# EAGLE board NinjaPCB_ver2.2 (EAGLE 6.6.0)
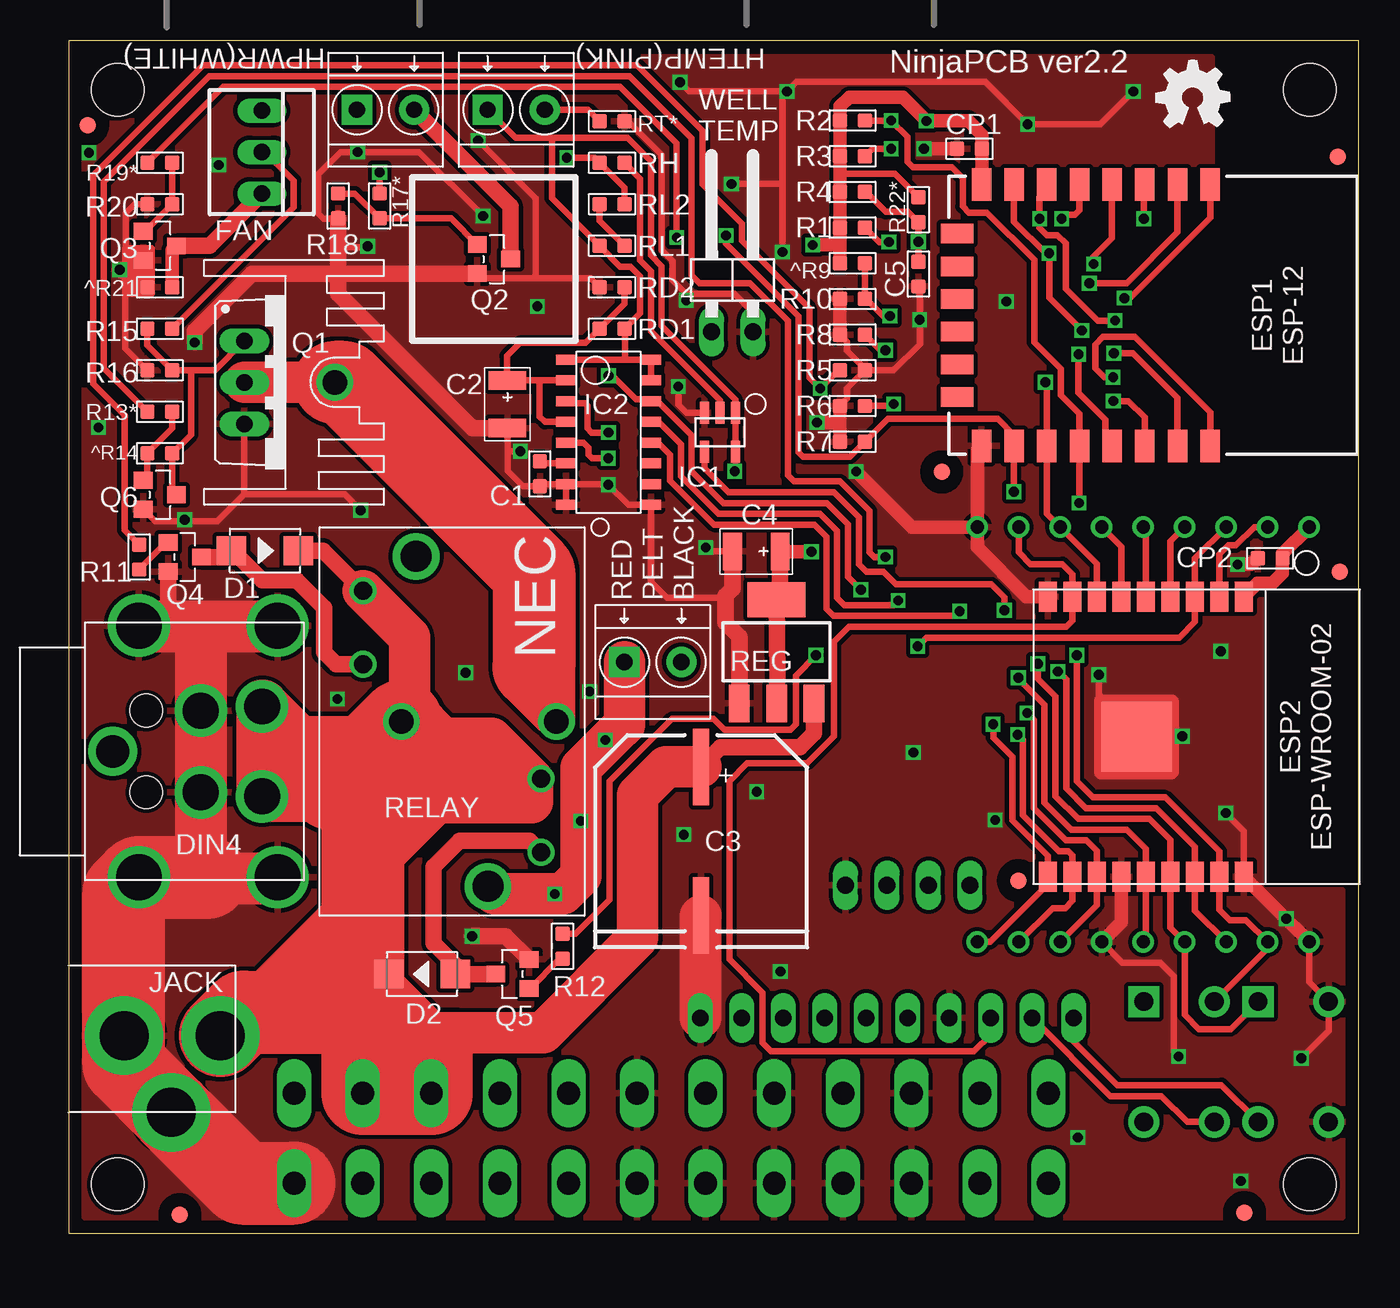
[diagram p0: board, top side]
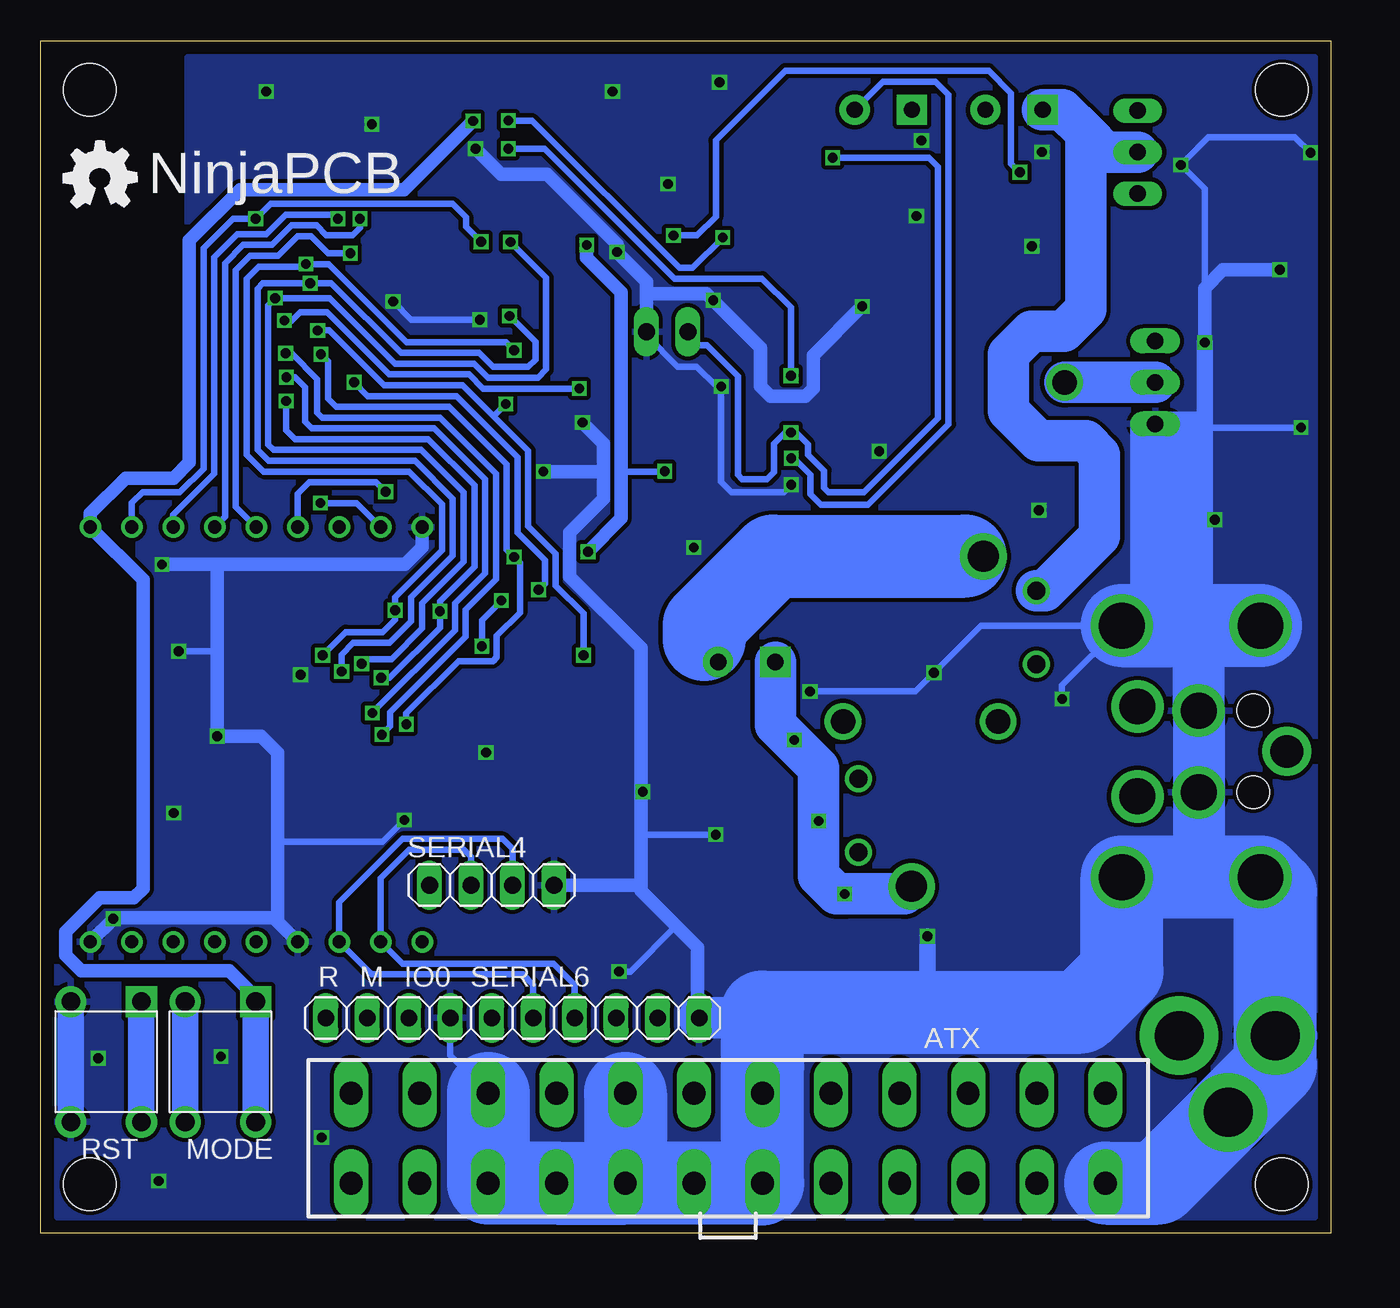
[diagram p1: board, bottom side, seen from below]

Size 79 x 73 mm. Coordinates in mm from the lower left corner, seen from the top.
Outline: 0,0 79,0 79,73 0,73 0,0
Copper layers (1*16): Top 0.035mm / dielectric 1.5mm / Bottom 0.035mm
Design rules "SeeedStudio_2oz": minimum track width 6mil, minimum drill 12mil, track to track 10mil, track to pad 10mil, pad to pad 10mil, via to via 10mil, smd to smd 0mil, copper to edge 10mil, drill to drill 10mil, minimum pad ring 10mil, minimum via ring 6mil, stop-mask expansion 2mil, vias tented up to drill 100mil, thermal gap 10mil
Net classes: 1 2A: width 0.406 mm; 2 8A: width 2.54 mm
Holes 3.2 mm at 3,3 3,70 76,70 76,3
tKeepout: area 1.4,1.4 to 4.6,4.6; area 74.4,1.4 to 77.6,4.6; area 74.4,68.4 to 77.6,71.6; area 1.4,68.4 to 4.6,71.6

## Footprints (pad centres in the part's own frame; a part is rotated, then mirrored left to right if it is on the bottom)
ATX24 = drill 1.4 long: 1 23.1,-2.75; 2 18.9,-2.75; 3 14.7,-2.75; 4 10.5,-2.75; 5 6.3,-2.75; 6 2.1,-2.75; 7 -2.1,-2.75; 8 -6.3,-2.75; 9 -10.5,-2.75; 10 -14.7,-2.75; 11 -18.9,-2.75; 12 -23.1,-2.75; 13 23.1,2.75; 14 18.9,2.75; 15 14.7,2.75; 16 10.5,2.75; 17 6.3,2.75; 18 2.1,2.75; 19 -2.1,2.75; 20 -6.3,2.75; 21 -10.5,2.75; 22 -14.7,2.75; 23 -18.9,2.75; 24 -23.1,2.75
C0603 = smd 0.889 x 0.889: 1 0,0.762; 2 0,-0.762
AVX-B = smd 1.143 x 2.286: + -1.46,0; - 1.46,0
CAP_SMD_AL_D125 = smd 1 x 4.7: P$M 0,-4.55; P$P 0,4.55
DO-214AC = smd 1.8 x 1.77: 1 -2.042,0; 2 2.042,0
DIN4 = drill 2.2: P$1 -2.75,10.85; P$2 2.75,10.85; P$3 -2.5,7.1; P$4 2.5,7.1 | drill 2: P$5 0,1.7 | drill 2.8: P$6 -7.7,11.8; P$7 -7.7,3.3; P$8 7.7,3.3; P$9 7.7,11.8 | hole 2: -2.5,3.75; 2.5,3.75
ESP-12F = smd 2 x 1.2: 1 -8,3.48; 2 -8,1.48; 3 -8,-0.52; 4 -8,-2.52; 5 -8,-4.52; 6 -8,-6.52; 7 -8,-8.52; 8 -8,-10.52; 15 8,-10.52; 16 8,-8.52; 17 8,-6.52; 18 8,-4.52; 19 8,-2.52; 20 8,-0.52; 21 8,1.48; 22 8,3.48 | smd 1.2 x 2: 9 -5,-12; 10 -3,-12; 11 -1,-12; 12 1,-12; 13 3,-12; 14 5,-12
ESP-WROOM-02 = smd 1.85 x 1.1: P$1 -8.575,12.9; P$2 -8.575,11.4; P$3 -8.575,9.9; P$4 -8.575,8.4; P$5 -8.575,6.9; P$6 -8.575,5.4; P$7 -8.575,3.9; P$8 -8.575,2.4; P$9 -8.575,0.9; P$10 8.575,0.9; P$11 8.575,2.4; P$12 8.575,3.9; P$13 8.575,5.4; P$14 8.575,6.9; P$15 8.575,8.4; P$16 8.575,9.9; P$17 8.575,11.4; P$18 8.575,12.9 | smd 4.3 x 4.3: P$19 0,6.33
ESP-WROOM-02-BREAK-NODETAIL = drill 0.8: P$1 -12.7,10.16; P$2 -12.7,7.62; P$3 -12.7,5.08; P$4 -12.7,2.54; P$5 -12.7,0; P$6 -12.7,-2.54; P$7 -12.7,-5.08; P$8 -12.7,-7.62; P$9 -12.7,-10.16; P$10 12.7,-10.16; P$11 12.7,-7.62; P$12 12.7,-5.08; P$13 12.7,-2.54; P$14 12.7,0; P$15 12.7,2.54; P$16 12.7,5.08; P$17 12.7,7.62; P$18 12.7,10.16
22-23-2031 = drill 1 long: 1 -2.54,0; 2 0,0; 3 2.54,0
H2-3.5-7.0X7.0MM = drill 1 pad 1.85 square: 1 -1.75,0 | drill 1 pad 1.85: 2 1.75,0
HEAT11PB015 = drill 1.5: P$1 0,3
SOT23-5 = smd 1.321 x 0.559: 1 -1.194,0.95; 2 -1.194,0; 3 -1.194,-0.95; 4 1.194,-0.95; 6 1.194,0.95
SOP-16 = smd 0.6 x 1.2: P$1 -4.445,-2.6; P$2 -3.175,-2.6; P$3 -1.905,-2.6; P$4 -0.635,-2.6; P$5 0.635,-2.6; P$6 1.905,-2.6; P$7 3.175,-2.6; P$8 4.445,-2.6; P$9 4.445,2.6; P$10 3.175,2.6; P$11 1.905,2.6; P$12 0.635,2.6; P$13 -0.635,2.6; P$14 -1.905,2.6; P$15 -3.175,2.6; P$16 -4.445,2.6
1X02 = drill 1.016 long: 1 -1.27,0; 2 1.27,0
PJ-102A-NOOUT = drill 3 pad 4.8: RING 0.1,-3.39; RING_SW -4.6,-6.29; TIP 0.1,-9.29
SW4-6.0X6.0X5.0MM = drill 1.143 pad 1.905 square: 1 -3.683,2.159 | drill 1.143 pad 1.905: 2 -3.683,-2.159; 3 3.683,-2.159; 4 3.683,2.159
TO220BV = drill 1.016 long: D 0,-2.54; G -2.54,-2.54; S 2.54,-2.54
SOT-23 = smd 1.016 x 1.143: 1 -0.889,-1.016; 2 0.889,-1.016; 3 0,1.016
R0603 = smd 0.889 x 0.889: 1 0,0.762; 2 0,-0.762
SOT-223 = smd 1.27 x 2.286: 1 -2.286,-3.175; 2 0,-3.175; 3 2.286,-3.175 | smd 3.556 x 2.159: TER 0,3.175
NEC-EP2 = drill 1.9: P$1 -10.1,-2.2; P$8 10.1,2.2 | drill 1.1: P$2 -8,-5.45; P$3 -3.5,-5.45; P$6 3.5,5.45; P$7 8,5.45 | drill 1.5: P$4 0,-3.1; P$5 0,6.4
1X04 = drill 1.016 long: 1 -3.81,0; 2 -1.27,0; 3 1.27,0; 4 3.81,0
1X06 = drill 1.016 long: 1 -6.35,0; 2 -3.81,0; 3 -1.27,0; 4 1.27,0; 5 3.81,0; 6 6.35,0
FIDUCIAL_1MM = smd 1 x 1: 1 0,0
1X02/90 = drill 1.016 long: 1 -1.27,-3.81; 2 1.27,-3.81

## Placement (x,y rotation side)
ATX  ATX24NH  [ATX24]  36.91,5.82 180 bottom
C1  100nf  [C0603]  28.86,46.49 180 top
C2  22uf  [AVX-B]  26.87,50.75 270 top
C3  CAP_SMDAL_1000UF_25V  [CAP_SMD_AL_D125]  38.73,24 0 top
C4  22uf  [AVX-B]  42.11,41.74 180 top
C5  100nf  [C0603]  52.04,58.72 180 top
CP1  100nf  [C0603]  55.16,66.4 270 top
CP2  100nf  [C0603]  73.57,41.32 90 top
D1  1N4007  [DO-214AC]  12.02,41.79 0 top
D2  1N4007  [DO-214AC]  21.64,15.88 180 top
DIN4  [DIN4]  1,29.5 270 top
ESP1  ESP-12F  [ESP-12F]  66.42,56.2 270 top
ESP2  ESP-WROOM-02  [ESP-WROOM-02]  59.08,30.4 270 top
ESP3  ESP-WROOM-02-BREAKND  [ESP-WROOM-02-BREAK-NODETAIL]  65.8,30.54 270 top
FAN  22-23-2031  [22-23-2031]  11.83,66.19 270 top
HEATER_POWER  [H2-3.5-7.0X7.0MM]  19.41,68.78 0 top
HEATER_TEMP  [H2-3.5-7.0X7.0MM]  27.41,68.78 0 top
HEATSINK  HEAT111PB015  [HEAT11PB015]  13.3,52.09 270 top
IC1  ANALOGSW_AD_SOT23-5  [SOT23-5]  39.88,49.04 270 top
IC2  NAU7802  [SOP-16]  33.06,49.04 270 top
IO0  [1X02]  55.19,13.18 0 bottom
JACK  2.1MMJACKTHM-NOOUT  [PJ-102A-NOOUT]  0,12 90 top
MODE  [SW4-6.0X6.0X5.0MM]  68,10.5 270 bottom
PELTIER  [H2-3.5-7.0X7.0MM]  35.77,34.97 0 top
Q1  IRLB3813PBF  [TO220BV]  13.3,52.09 270 top
Q2  CJ2302  [SOT-23]  26.04,59.63 270 top
Q3  CJ2302  [SOT-23]  5.59,60.45 270 top
Q4  S9013  [SOT-23]  7.11,41.4 270 top
Q5  S9013  [SOT-23]  27.18,15.88 90 top
Q6  S9013  [SOT-23]  5.59,45.21 270 top
R1  10K 1/10W  [R0603]  48.01,61.57 90 top
R2  10K 1/10W  [R0603]  48.01,68.12 90 top
R3  10K 1/10W  [R0603]  48.01,65.94 90 top
R4  10K 1/10W  [R0603]  48.01,63.75 90 top
R5  10K 1/10W  [R0603]  48.01,52.83 270 top
R6  10K 1/10W  [R0603]  48.01,50.65 90 top
R7  10K 1/10W  [R0603]  48.01,48.46 90 top
R8  10K 1/10W  [R0603]  48.01,55.02 90 top
R9  100K 1/10W  [R0603]  48.01,59.39 270 top
R10  10K 1/10W  [R0603]  48.01,57.2 270 top
R11  10K 1/10W  [R0603]  4.32,41.4 0 top
R12  10K 1/10W  [R0603]  30.25,17.58 180 top
R13  1K 1/10W  [R0603]  5.59,50.29 90 top
R14  0R  [R0603]  5.59,47.75 90 top
R15  10K 1/10W  [R0603]  5.59,55.37 90 top
R16  10K 1/10W  [R0603]  5.59,52.83 90 top
R17  1K 1/10W  [R0603]  19.05,62.89 0 top
R18  10K 1/10W  [R0603]  16.51,62.89 180 top
R19  1K 1/10W  [R0603]  5.59,65.53 90 top
R20  10K 1/10W  [R0603]  5.59,62.99 90 top
R21  0R  [R0603]  5.59,57.91 90 top
R22  1K 1/10W  [R0603]  52.04,62.66 180 top
RD1  15K HP  [R0603]  33.27,55.37 90 top
RD2  15K HP  [R0603]  33.27,57.91 270 top
REG  CJT1117-3.3-SOT223  [SOT-223]  43.36,35.61 0 top
RELAY  NEC-RELAY2EP2  [NEC-EP2]  23.48,31.34 270 top
RESET  [1X02]  60.27,13.18 0 bottom
RH  15K HP  [R0603]  33.27,65.53 270 top
RL1  15K HP  [R0603]  33.27,60.45 90 top
RL2  15K HP  [R0603]  33.27,62.99 90 top
RST  [SW4-6.0X6.0X5.0MM]  75,10.5 270 bottom
RT  4.99K HP  [R0603]  33.27,68.07 90 top
SERIAL4  [1X04]  51.38,21.31 0 bottom
SERIAL6  [1X06]  45.03,13.18 0 bottom
U$1  [OSHW_5MM]  68.83,69.52 0 top
U$2  [OSHW_5MM]  75.39,64.59 0 bottom
U$3  FIDUCIAL  [FIDUCIAL_1MM]  77.72,65.91 270 top
U$4  FIDUCIAL  [FIDUCIAL_1MM]  6.81,1.14 0 top
U$5  FIDUCIAL  [FIDUCIAL_1MM]  72.01,1.27 0 top
U$7  FIDUCIAL  [FIDUCIAL_1MM]  1.17,67.84 0 top
U$8  FIDUCIAL  [FIDUCIAL_1MM]  58.17,21.59 270 top
U$9  FIDUCIAL  [FIDUCIAL_1MM]  53.47,46.61 270 top
U$10  FIDUCIAL  [FIDUCIAL_1MM]  77.85,40.51 270 top
WELL_TEMP  [1X02/90]  40.64,59 0 top

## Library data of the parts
ATX DIN4 HEATSINK = PCR-Connector
C1 C5 CP1 CP2 = Seeed-Capacitor; MPN: CC0603KRX7R9BB104
C2 C4 = Seeed-Capacitor; MPN: TAJB226*016#NJ
C3 = Seeed-OPL-2017-01-Capacitor-akita
D1 D2 = Seeed-Diode; MPN: 1N4007
ESP1 = Seeed-OPL-2017-01-Sensor-camilo
ESP2 ESP3 = PCR-Module
FAN = con-molex; MF: MOLEX; MPN: 22-23-2031; OC_FARNELL: 1462950; OC_NEWARK: 30C0862
HEATER_POWER HEATER_TEMP PELTIER = Seeed-Connector
IC1 IC2 = PCR-IC
IO0 RESET SERIAL4 SERIAL6 WELL_TEMP = pinhead
JACK U$3-U$5 U$7-U$10 = adafruit
MODE RST = Seeed-Switch
Q1 = transistor-power
Q2 Q3 = Seeed-Transistor; MPN: CJ2302
Q4-Q6 = Seeed-Transistor; MPN: S9013
R1-R8 R10-R12 R15 R16 R18 R20 = Seeed-Resistor; MPN: RC0603JR-0710KL
R9 = Seeed-Resistor; MPN: RC0603JR-07100KL
R13 R17 R19 R22 = Seeed-Resistor; MPN: RC0603JR-071KL
R14 R21 = Seeed-Resistor; MPN: RC0603JR-070RL
RD1 RD2 RH RL1 RL2 = PCR-RCL
REG = Seeed-IC; MPN: CJT1117-3.3
RELAY = PCR-Switch
RT = Seeed-Resistor; MPN: RC0603FR-072KL
U$1 U$2 = oshw

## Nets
3V3: C4.+ CP1.1 CP2.2 ESP1.8 ESP2.P$1 ESP3.P$1 HEATER_TEMP.1 IC1.1 IC1.6 IC2.P$1 IC2.P$15 IC2.P$16 MODE.1 MODE.4 R1.1 R2.1 R3.1 R4.1 R9.2 R22.2 RD1.2 REG.2 REG.TER RL1.1
12V: ATX.10 ATX.11 C3.P$P D1.2 D2.2 DIN4.P$1 DIN4.P$2 FAN.2 HEATER_POWER.1 JACK.TIP R15.2 REG.3 RELAY.P$2 RELAY.P$4 RELAY.P$6
BLK: PELTIER.2 RELAY.P$1
DIVIDED: C2.+ IC2.P$2 IC2.P$4 RD1.1 RD2.1
DRDY: ESP1.20 ESP2.P$14 ESP3.P$14 IC2.P$12
EN: C5.2 ESP1.3 ESP2.P$2 ESP3.P$2 R4.2 R22.1
FAN: ESP1.18 ESP2.P$8 ESP3.P$8 IO0.1 R2.2 R19.1
GND: ATX.3 ATX.5 ATX.7 ATX.15 ATX.16 ATX.17 ATX.18 ATX.19 ATX.24 C1.1 C2.- C3.P$M C4.- C5.1 CP1.2 CP2.1 DIN4.P$3 DIN4.P$4 DIN4.P$6 DIN4.P$7 DIN4.P$8 DIN4.P$9 ESP1.15 ESP2.P$9 ESP2.P$13 ESP2.P$18 ESP2.P$19 ESP3.P$9 ESP3.P$13 ESP3.P$18 IC1.3 IC2.P$7 IC2.P$8 IC2.P$9 IO0.2 JACK.RING JACK.RING_SW Q1.S Q2.2 Q3.2 Q4.2 Q5.2 Q6.2 R5.1 R6.1 R7.1 R8.1 R10.2 R16.1 R18.1 R20.1 R21.1 RD2.2 REG.1 RST.2 RST.3 RT.2 SERIAL4.4 SERIAL6.6 WELL_TEMP.2
HEATER: ESP1.16 ESP2.P$6 ESP3.P$6 R7.2 R17.1
HEATER_TEMP: HEATER_TEMP.2 IC2.P$5 RT.1
HIGH_TEMP: ESP1.4 ESP2.P$17 ESP3.P$17 IC1.4 MODE.2 MODE.3 R8.2 RESET.2
N$1: RL1.2 RL2.1
N$2: HEATER_POWER.2 Q2.3
N$3: HEATSINK.P$1 Q1.D RELAY.P$5
N$4: FAN.3 Q3.3 R21.2
N$5: Q1.G Q6.3 R14.2 R15.1 R16.2
N$8: Q3.1 R19.2 R20.2
N$27: IC1.2 RH.1
N$30: Q6.1 R13.2 R14.1
N$32: Q2.1 R17.2 R18.2
N$33: D1.1 Q4.3 RELAY.P$3
N$34: Q4.1 R11.2
N$35: Q5.1 R12.1
N$36: D2.1 Q5.3 RELAY.P$7
N$92: C1.2 IC2.P$6
PEL_PWM: ESP1.19 ESP2.P$10 ESP3.P$10 R13.1
PEL_SWA: ESP1.6 ESP2.P$4 ESP3.P$4 R5.2 R11.1
PEL_SWB: ESP1.7 ESP2.P$5 ESP3.P$5 R6.2 R12.2
RED: PELTIER.1 RELAY.P$8
RESET: ESP1.1 ESP2.P$15 ESP3.P$15 R1.2 RESET.1 RST.1 RST.4
RXD: ESP1.21 ESP2.P$11 ESP3.P$11 SERIAL4.2 SERIAL6.3
SCLK: ESP1.5 ESP2.P$3 ESP3.P$3 IC2.P$13
SDIO: ESP1.17 ESP2.P$7 ESP3.P$7 IC2.P$14 R3.2
TOUT: ESP1.2 ESP2.P$16 ESP3.P$16 R9.1 R10.1
TXD: ESP1.22 ESP2.P$12 ESP3.P$12 SERIAL4.3 SERIAL6.2
WELL_TEMP: IC2.P$3 RH.2 RL2.2 WELL_TEMP.1

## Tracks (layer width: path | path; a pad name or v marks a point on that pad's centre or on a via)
3V3  (via drill 0.6)
  Top 0.406: IC2.P$1 34.09,53.48 | 34.09,53.48 IC2.P$16 IC2.P$15 | 34.09,53.48 34.09,55.32 RD1.2 35,56.34 35,58.6 34.42,59.18 33.78,59.18 RL1.1 29.59,63.37 29.59,67.08 | HEATER_TEMP.1 27.36,67.08 29.59,67.08 | 29.59,67.08 34.21,67.08 35.66,65.63 35.66,59.87 36.32,59.21 36.32,55.55 40.83,51.04 IC1.1 IC1.6 40.83,46.66 v40.79,46.66 | R22.2 50.6,64.87 47.24,64.87
  Top 0.813: 43.35,34.1 43.41,34.16 | C4.+ 43.66,41.73 v45.49,41.73 | ESP1.8 55.93,64.2 CP1.1 55.93,67.26 55.09,68.1 v52.53,68.1 51.08,69.55 47.8,69.55 47.24,68.99 R2.1 R3.1 47.24,64.87 R4.1 R1.1 47.24,60.5 | ESP2.P$1 72.8,39.8 73.71,39.8 74.31,40.4 CP2.2 74.34,41.61 ESP3.P$1 | v45.57,60.5 47.24,60.5 | R9.2 47.24,60.5
  Top 1.016: REG.2 43.41,34.16 REG.TER 43.58,39.01 C4.+
  Bottom 0.406: 45.49,41.83 v45.49,41.73 | v40.79,46.66 40.82,46.63 43.46,46.63
  Bottom 0.813: v45.49,41.73 43.46,43.76 43.46,46.63 43.46,57.61 45.57,59.72 v45.57,60.5 | MODE.1 65.84,14.46 67.46,16.08 76.53,16.08 77.47,17.02 77.47,18.47 75.39,20.55 73.3,20.55 72.75,21.11 72.75,40.02 ESP3.P$1 75.96,44.08 73.81,46.23 70.87,46.23 69.9,47.19 69.9,60.78 66.8,63.88 56.74,63.88 v52.53,68.1
  Bottom 1.626: MODE.4 MODE.1
12V
  Top 0.254: 28.37,27.84 28.36,27.84 28.36,27.85 | 19.25,15.21 20.4,15.21 20.4,12.29 | 17.2,20.02 18.01,20.02 18.01,20.24
  Top 0.406: FAN.2 12.05,66.19 13.79,64.44 13.79,62.81 R15.2 | DIN4.P$1 11.86,32.26 | 23.5,8.56 22.22,8.56 ATX.10
  Top 0.508: 16.05,27.23 16.48,27.23 16.71,27.46
  Top 1.016: RELAY.P$2 15.58,41.79 D1.2 | D2.2 19.53,15.74 17.32,13.54 17.5,13.36 17.5,12.9 18.01,12.39 ATX.11 | REG.3 45.65,30.61 44.78,29.74 39.91,29.74 C3.P$P
  Top 1.27: 28.37,27.84 RELAY.P$6
  Top 2.54: RELAY.P$2 20.88,36.49 20.88,32.21 20.38,31.71 RELAY.P$4 23.88,27.84 28.37,27.84 | 23.72,12.29 23.5,12.06 23.5,8.56 | 23.72,12.29 20.4,12.29 | 23.72,12.29 29.06,12.29 34.85,18.09 34.85,26.82 36.58,28.55 C3.P$P | 18.62,20.75 18.62,22.45 23.39,27.23 21.06,27.23 20.75,26.92 20.75,27.64 21.34,28.22 23.19,26.36 28.35,26.36 28.4,26.42 28.4,27.81 28.36,27.85 25.91,30.3 22.91,30.3 21.08,32.13 20.73,32.13 19,30.4 14.02,30.4 | 19.25,21.39 19.25,15.21 21.89,12.57 | 17.2,23.27 17.2,20.02 12.06,14.88 14.55,14.88 15.6,15.93
  Top 3.175: 15.36,26.75 DIN4.P$2 DIN4.P$1 | 11.89,32.23 11.86,32.26 11.86,32.31 16.71,27.46 | 13.01,28.73 13.56,28.17 14.15,28.17
  Top 5.08: ATX.10 ATX.11 18.01,20.24 18.01,26.16 16.71,27.46 | RELAY.P$4 16.27,27.23 16.05,27.23 15.11,28.17 14.15,28.17 | JACK.TIP 10.73,13.54 17.32,13.54 17.45,13.54
  Bottom 2.54: 15.01,67.36 15.01,56.57 16.36,55.22 18.34,55.22 19.74,53.82 19.74,50.34 17.91,48.51 15.01,48.51 14.17,47.68 14.17,42.67 17.51,39.34 RELAY.P$2 | 15.01,67.36 16.43,68.78 HEATER_POWER.1 | 15.01,67.36 13.84,66.19 FAN.2
BLK
  Bottom 0.508: 38.38,36.35 37.52,35.49 PELTIER.2 | 22.4,41.45 22.39,41.44 RELAY.P$1
  Bottom 5.08: 38.38,36.35 38.38,37.24 34.16,41.45 22.4,41.45
DIVIDED
  Top 0.406: IC2.P$2 28.8,52.21 | 28.8,52.21 C2.+ 26.85,52.24 26.85,53.72 27.64,54.51 31.65,54.51 RD1.1 34.04,56.9 RD2.1 | IC2.P$4 29.17,49.67 28.85,49.99 28.85,52.16 28.8,52.21
DRDY  (via drill 0.6)
  Top 0.406: IC2.P$12 36.1,48.4 36.83,47.68 36.83,46.08 39.52,43.38 45.67,43.38 46.41,42.65 46.41,38.23 46.84,37.8 54.28,37.8 v54.56,38.08 | ESP3.P$14 65.98,18.01 ESP2.P$14 65.98,23.53 64.8,24.71 61.42,24.71 59.77,26.36 59.77,32.36 58.17,33.96 v58.17,34.01 | ESP1.20 65.9,49.95 64.9,50.95 v63.98,50.95
  Bottom 0.406: v63.98,50.95 63.98,49.17 63.42,48.62 55.27,48.62 52.45,45.8 52.45,40.79 54.56,38.68 v54.56,38.08 54.56,37.08 57.63,34.01 v58.17,34.01
EN  (via drill 0.6)
  Top 0.406: ESP2.P$2 70.48,41.57 71.02,42.11 71.48,42.11 72.6,43.24 ESP3.P$2 | ESP1.3 65.84,64.14 v65.84,62.1 | R4.2 48.82,63.75 50.04,62.53 51.41,62.53 R22.1 v52.05,60.69 C5.2
  Bottom 0.406: ESP3.P$2 73.42,44.71 72.77,45.36 70.48,45.36 69.04,46.81 69.04,60.3 67.23,62.1 v65.84,62.1 64.92,63.02 53.77,63.02 52.96,62.2 52.96,61.61 v52.05,60.69
FAN  (via drill 0.6)
  Top 0.406: R19.1 9.47,70.18 33.78,70.18 37.24,66.73 v37.24,60.96 | ESP3.P$8 58.18,41.69 58.9,40.97 60.86,40.97 61.48,40.35 ESP2.P$8 61.48,37.5 61.11,37.13 47.78,37.13 46.86,36.22 46.86,30.43 45.21,28.78 41.55,28.78 40.46,27.69 40.46,16.76 42.49,14.73 42.49,11.66 43,11.15 55.45,11.15 56.46,12.17 IO0.1 | v61.87,44.7 61.9,44.73 ESP1.18 61.9,50.16 60.76,51.31 60.76,52.93 59.13,54.56 59.13,59.59 56.24,62.48 55.14,62.48 54.76,62.87 54.76,64.59 54.1,65.25 51.71,65.25 51.36,65.61 51.36,67.13 v50.37,68.12 R2.2
  Bottom 0.406: ESP3.P$8 59.65,44.7 v61.87,44.7 | v37.24,60.96 39.09,59.11 39.9,59.11 48.92,68.12 v50.37,68.12
GND  (via drill 0.6)
  Top 0.406: Q6.2 5.31,43.59 7.01,43.59 | 7.01,43.59 9.09,43.59 10.76,45.26 | 10.76,45.26 Q1.S | 4.83,59.31 Q3.2 | R20.1 4.04,62.99 3.5,62.46 3.5,60.33 | 4.29,59.56 Q3.2 | 3.5,60.33 4.06,59.77 4.37,59.77 Q3.2 | R21.1 4.8,57.91 4.78,57.89 | 5.08,58.42 5.08,57.53 3.48,57.53 | 3.48,57.53 3.48,60.3 | 3.48,60.3 3.76,60.3 3.76,59.38 3.79,59.38 3.79,60.3 5.08,60.3 5.08,59.74 4.01,59.74 4.01,60.07 4.57,60.07 4.57,60.05 | IC2.P$8 IC2.P$7 | IC2.P$7 28.99,45.86 C1.1 27.83,45.73 26.87,46.69 26.87,47.88 | 26.87,47.88 C2.- | RD2.2 31.95,58.47 28.6,58.47 | 28.6,58.47 25.3,58.47 Q2.2 | IC2.P$7 33,45.86 v33.05,45.82 34.27,44.59 IC2.P$9 35.66,39.9 36.65,38.91 40.11,38.91 40.23,39.04 | v37.34,51.84 37.34,51.33 37.34,50.93 37.34,50.72 37.83,50.23 IC1.3 | RT.2 34.27,68.07 36.32,66.02 36.32,60.2 36.98,59.54 36.98,58.34 37.82,57.51 38.1,57.51 | 38.1,57.51 40.77,57.51 41.91,56.36 WELL_TEMP.2 | ESP3.P$18 75.96,15.38 RST.2 77.16,12.39 v75.49,10.72 | 4.32,21.79 5.49,21.79 5.56,21.72 | 63.25,28.19 65.96,28.19 v68.2,30.43 | 3.76,58.75 3.66,58.75 | 3.48,60.3 3.5,60.33 | 47.24,57.05 R10.2 | v18.31,60.43 18.26,60.38 16.51,60.38 | v43.99,69.9 43.71,69.62 43.71,64.24 | 43.71,64.24 v43.71,60.07 | v43.99,69.9 44.58,70.48 56.13,70.48 v58.73,67.89 63.2,67.89 v65.2,69.9 | v70.87,25.73 71.98,24.62 ESP2.P$18 | v63.09,34.19 63.09,32.31 64.19,31.22 64.59,31.22 ESP2.P$19 | v17.88,44.27 16.9,45.26 10.76,45.26 | v40.59,64.24 43.71,64.24 | v74.57,19.25 74.55,19.25 74.05,19.75 | v37.82,57.12 37.82,57.23 38.1,57.51 | R18.1 16.48,62.1 15.62,62.1 15.29,62.43 15.29,64.82 16.66,66.19 v17.7,66.19 21.46,66.19 v25.38,62.28 | v25.07,66.9 28.6,63.37 28.6,58.47
  Top 0.406: v27.66,47.88 26.87,47.88 | v39.01,41.99 39.26,41.74 C4.- | 7.01,43.59 v7.11,43.69 | v43.99,69.9 38,69.9 v37.44,70.46 | R16.1 3.48,54.18 3.48,57.53 | v67.97,10.82 67.67,11.12 67.67,15.75 66.85,16.56 64.54,16.56 ESP3.P$13 | R5.1 48.77,52.93 47.68,54.03 47.68,54.59 R8.1 | R6.1 47.68,51.08 47.68,51.74 R5.1 | R5.1 50.52,52.83 52.12,54.43 v52.12,55.93 52.12,57.89 C5.1
  Top 0.813: 4.78,57.89 3.96,57.89 3.66,58.19 3.66,58.75 4.19,58.22 4.88,58.22 4.67,58.42 4.67,59.08 4.88,58.88 | 4.88,58.88 4.88,58.29 | 4.88,58.88 4.88,59.82 | ESP2.P$9 58.66,38.98 55.64,41.99 ESP3.P$9 | CP2.1 72.43,40.95 v71.58,40.95 | ESP2.P$19 68.17,30.4 v68.2,30.43 | ESP2.P$13 64.48,19.05 ESP3.P$13 | ESP2.P$18 74.05,19.75 ESP3.P$18 | 63.25,32.59 63.27,32.56 67.56,32.56 67.59,32.54 67.59,28.25 67.54,28.19 63.25,28.19 63.22,28.22 63.22,32.59 | ESP3.P$9 55.64,47.94 ESP1.15 | v48.23,46.63 51.63,43.24 ESP3.P$9 | 47.14,57.2 R10.2 R8.1 | R7.1 47.24,49.84 | 47.24,49.84 R6.1 | v45.82,49.63 47.04,49.63 47.24,49.84 | CP1.2 v52.38,66.39 v52.38,66.4
  Top 1.016: 4.47,37.13 4.41,37.2 DIN4.P$7 5.51,37.2 6.1,37.78 Q4.2 | v3.12,58.98 3.76,58.75 Q3.2 | Q2.2 16.43,58.75 | 16.43,58.75 11.25,58.75 7.72,55.22 v7.72,54.53 | R18.1 16.51,60.38 16.51,58.82 | 16.51,58.82 16.43,58.75 | C2.- 24.75,49.29 16.51,57.53 16.51,58.82 | v24.71,18.19 26.77,18.19 Q5.2 | REG.1 41.07,36.52 40.23,37.36 40.23,39.04 40.65,39.46 C4.-
  Top 2.54: C3.P$M 38.68,19.41 SERIAL6.6
  Top 3.175: 4.19,21.77 4.24,21.72 5.56,21.72 8.1,21.72 | 12.72,21.72 8.1,21.72 | 8.1,21.72 8.1,37.13 4.47,37.13 4.24,37.13 4.24,37.16 12.85,37.16
  Top 5.08: 4.12,21.61 DIN4.P$8 4.32,21.79 | 4.32,21.79 8.46,21.79 | 4.32,21.79 3.38,20.85 3.38,10.34 6.29,7.43 JACK.RING_SW 10.62,3.07 ATX.24
  Bottom 0.254: 11.02,49.02 12.17,49.02 12.17,49.58 10.76,49.58 | 10.76,49.58 Q1.S | 9.63,49.58 10.76,49.58
  Bottom 0.406: WELL_TEMP.2 41.91,54.97 40.01,53.06 38.84,53.06 37.62,51.84 v37.34,51.84 37.34,46 36.7,45.36 33.5,45.36 v33.05,45.82 | IO0.2 53.92,10.89 ATX.3 | ATX.7 34.8,8.58 34.8,10.24 | 13.79,3.07 ATX.24 | v7.72,54.53 7.72,63.93 v9.2,65.41 7.49,67.11 2.21,67.11 v1.25,66.14 | v70.56,35.64 68.56,35.64 68.2,35.99 | v1.83,49.33 7.7,49.33 7.8,49.23 | v37.67,24.41 42.24,24.41 | v42.14,27.03 42.14,26.98 42.24,26.87 | v31.9,33.17 25.45,33.17 v24.31,34.31 21.42,37.2 DIN4.P$6 16.46,33.54 v16.46,32.72 | v43.59,16.03 42.9,16.03 40.09,18.83 | 64.49,23.98 58.06,23.98 v56.74,25.3 | v52.12,55.93 56.31,55.93 v57.43,57.05
  Bottom 0.813: v71.58,40.95 68.38,40.95 | 68.38,40.95 56.69,40.95 55.64,41.99 ESP3.P$9 | 68.38,40.95 68.2,40.77 68.2,35.99 v68.2,30.43 65.51,30.43 64.49,29.41 64.49,23.98 64.49,19.07 | ESP3.P$13 64.49,19.07 | 64.49,19.07 64.75,19.33 74.47,19.33 ESP3.P$18 | 44.53,46.81 44.53,44.98 46.61,42.9 46.61,40.21 42.24,35.84 42.24,26.87 42.24,24.41 42.24,21.31 | v48.23,46.63 44.65,46.63 44.53,46.81 | WELL_TEMP.2 41.91,57.68 | 41.91,57.68 41.91,58.27 v43.71,60.07 43.71,60.55 48.01,64.85 50.83,64.85 v52.38,66.4 | 34.8,3.07 ATX.19 35.2,3.47 35.2,12.9 35.46,13.16 38.71,13.16 38.79,13.23 38.79,17.53 40.09,18.83 42.24,20.98 42.24,21.31 | SERIAL4.4 42.24,21.31 | v28.7,56.74 31.7,53.75 31.7,51.74 32.18,51.26 34.31,51.26 34.92,51.87 34.92,54.2 38.23,57.51 41.73,57.51 41.91,57.68 | v7.72,54.53 7.72,57.86 6.6,58.98 v3.12,58.98 | 44.53,46.81 44.53,48.34 v45.82,49.63
  Bottom 1.016: 9.63,49.58 7.72,47.68 | v7.72,54.53 7.72,46.94 8.48,47.7 8.48,49.23 10.44,49.23 Q1.S 10.62,49.7 10.62,49.81 7.8,49.81 7.8,49.23 7.8,48.74 | v24.71,18.19 24.71,13.54
  Bottom 1.626: RST.2 RST.3
  Bottom 2.54: 9.75,47.78 11.02,47.78 11.02,49.02 | SERIAL6.6 34.81,13.18
  Bottom 3.175: DIN4.P$8 8.1,21.8 DIN4.P$4 DIN4.P$3 8.1,37.2 DIN4.P$7
  Bottom 5.08: ATX.17 ATX.18 ATX.19 | 3.39,10.3 JACK.RING 3.39,20.89 DIN4.P$8 DIN4.P$9 12.8,16.05 15.32,13.54 24.71,13.54 34.81,13.54 34.81,13.18 ATX.7 | DIN4.P$7 DIN4.P$6 9.75,37.2 9.75,47.78 | ATX.17 ATX.16 ATX.15 ATX.3 | 13.79,3.07 10.59,3.07 3.43,10.24 | 34.85,3.02 34.8,3.07 34.8,10.24 | ATX.5 ATX.17
  other vias: 71.78,3.2 51.74,29.44 61.8,5.87
  pour Top (isolate 0.254): 1,72 70,72 70,48 73,48 73,21 78,21 78,1 1,1
  pour Bottom (isolate 0.254): 1,72 70,72 70,48 73,48 73,21 78,21 78,1 1,1
HEATER  (via drill 0.6)
  Top 0.406: R17.1 v19.05,64.95 | ESP3.P$6 64.48,42.03 ESP2.P$6 | v57.89,45.39 57.89,48.19 ESP1.16 57.9,48.86 56.9,49.86 50.16,49.86 R7.2 47.85,47.55 44.98,47.55 44.7,47.83 44.7,56.13 40.26,60.58 v40.26,61.09
  Bottom 0.406: v19.05,64.95 19.58,65.48 19.58,69.8 20.95,71.17 33.4,71.17 37.67,66.9 37.67,62.23 38.81,61.09 v40.26,61.09 | ESP3.P$6 63.26,45.27 62.56,45.97 58.47,45.97 v57.89,45.39
HEATER_TEMP  (via drill 0.6)
  Top 0.406: 30.48,48.39 IC2.P$5 31.53,48.4 31.85,48.08 31.85,47.65 32.05,47.45 v33.05,47.45 | RT.1 31.8,68.78 HEATER_TEMP.2
  Bottom 0.406: HEATER_TEMP.2 27.43,70.51 24.23,70.51 23.42,69.7 23.42,49.53 28.35,44.6 31.24,44.6 31.88,45.24 31.88,46.43 32.89,47.45 v33.05,47.45
HIGH_TEMP  (via drill 0.6)
  Top 0.406: MODE.3 68.49,6.82 66.9,8.41 63.78,8.41 RESET.2 | MODE.2 73.42,17.45 ESP3.P$17 72.09,19.18 71.09,19.18 70.48,19.8 ESP2.P$17 70.48,23.38 67.16,26.7 62.71,26.7 61.75,27.66 v61.75,35.38 | v57.3,38.15 57.3,38.94 56.52,39.73 50.65,39.73 49.89,40.49 48.87,40.49 48.39,40.97 48.39,43.84 46.86,45.36 40.41,45.36 38.93,46.84 IC1.4 | ESP1.4 63.9,60.93 62.76,59.79 v62.76,59.33 | R8.2 48.79,54.99 48.79,54.97 49.71,54.05 v50.01,54.05
  Bottom 0.406: v61.75,35.38 60.33,36.8 58.06,36.8 57.3,37.57 v57.3,38.15 57.3,38.94 54.43,41.81 54.43,44.63 56.44,46.63 65.35,46.63 66.4,47.68 66.4,58.45 65.66,59.18 62.92,59.18 v62.76,59.33 61.37,59.33 56.59,54.56 50.52,54.56 v50.01,54.05
  Bottom 1.626: MODE.3 MODE.2
N$1
  Top 0.406: RL1.2 32.51,61.98 RL2.1
N$2
  Top 1.016: HEATER_POWER.2 27.06,62.88 Q2.3
N$3
  Top 0.406: Q1.D
  Top 1.27: 28.5,34.67 30.4,34.67 30.4,31.32 29.13,31.32 27.13,33.33 28.5,33.33 29.64,32.18 29.64,31.58 RELAY.P$5
  Top 2.54: Q1.D 16.18,52.09
  Top 5.08: HEATSINK.P$1 16.84,52.09 28.5,40.44 28.5,34.67
  Bottom 2.54: Q1.D HEATSINK.P$1
N$4
  Top 0.813: R21.2 6.35,60.2 Q3.3
  Top 1.016: FAN.3 8.63,60.45 Q3.3
N$5
  Top 0.406: Q6.3 6.35,45.47 R14.2 7.49,48.9 7.49,52.83 | Q1.G 8.96,52.83 7.49,52.83 | 7.49,52.83 R16.2 4.83,54.36 R15.1
N$8
  Top 0.406: Q3.1 4.7,61.34 R20.2 R19.2
N$27
  Top 0.406: RH.1 35,64.57 35,59.56 35.66,58.9 35.66,55.22 39.88,51 IC1.2
N$30
  Top 0.406: Q6.1 4.83,46.35 R14.1 6.35,49.28 R13.2
N$32
  Top 0.406: R18.2 17.53,63.65 R17.2 23.42,62.13 Q2.1
N$33
  Top 1.016: RELAY.P$3 16.37,34.84 15.65,35.56 15.65,38.3 13.97,39.98 11.86,39.98 10.05,41.79 D1.1 9.59,41.4 Q4.3
N$34
  Top 0.406: Q4.1 5.97,42.29 R11.2
N$35
  Top 0.406: Q5.1 28.25,14.99 30.07,16.82 R12.1
N$36
  Top 1.016: D2.1 23.39,16.18 | D2.1 Q5.3 | 23.47,15.88 D2.1 | RELAY.P$7 28.24,24.03 23.95,24.03 22.35,22.43 22.35,17.75 23.68,16.42 D2.1
N$92
  Top 0.406: IC2.P$6 28.98,47.13 C1.2
PEL_PWM  (via drill 0.6)
  Top 0.406: R13.1 2.16,52.96 2.16,64.39 2.69,64.92 2.79,65.02 8.61,70.84 34.34,70.84 38.15,67.03 38.15,58.65 38.63,58.17 41.73,58.17 44.04,55.85 44.04,46.41 44.42,46.02 47.24,46.02 49.05,44.22 49.05,41.71 49.35,41.4 v50.01,41.4 | ESP3.P$10 56.45,17.84 59.98,21.37 ESP2.P$10 59.98,23.11 57.78,25.3 57.78,29.18 56.62,30.35 v56.62,31.17 | ESP1.19 63.9,48.77 63.5,49.17 63.5,49.81 61.85,51.46 v61.85,53.82
  Bottom 0.406: v61.85,53.82 61.42,53.39 61.42,51.1 60.91,50.6 54,50.6 50.47,47.07 50.47,41.86 v50.01,41.4 49.66,41.05 49.66,38 51.08,36.58 51.08,35.26 51.31,35.03 53.42,35.03 56.62,31.83 v56.62,31.17
PEL_SWA  (via drill 0.6)
  Top 0.406: R11.1 3.43,43.05 3.43,50.09 1.5,52.02 1.5,64.77 8.23,71.5 34.8,71.5 38.81,67.49 38.81,64.21 41.22,61.8 41.22,60.76 45.36,56.62 45.36,52.38 v46.02,51.71 47.14,52.83 R5.2 | ESP3.P$4 67.48,42.37 ESP2.P$4 | v64.08,55.88 63.02,55.88 61.06,57.84 61.06,60.6 60.55,61.11 59.92,61.11 59.46,61.57 v59.46,62.1 59.46,63.41 59.9,63.85 ESP1.6
  Bottom 0.406: ESP3.P$4 67.72,43.87 67.72,59.38 66.6,60.5 64.82,60.5 63.63,61.7 62.1,61.7 61.52,61.11 59.92,61.11 59.46,61.57 v59.46,62.1 | v64.08,55.88 63.63,55.88 63.12,56.39 61.47,56.39 57.66,52.58 52.78,52.58 51.92,51.71 v46.02,51.71
PEL_SWB  (via drill 0.6)
  Top 0.406: ESP3.P$5 65.98,43.07 ESP2.P$5 | R12.2 31.04,18.34 33.12,20.42 33.12,27.66 36.96,31.5 39.5,31.5 40.16,30.84 44.2,30.84 44.53,31.17 44.53,34.14 v45.77,35.38 | ESP1.7 57.9,61.94 59.84,59.99 v60.05,59.99 60.05,57.28 v62.05,55.27 | R6.2 50.39,50.65 v50.52,50.77
  Bottom 0.406: ESP3.P$5 67.06,44.49 67.06,58.95 66.17,59.84 64.47,59.84 63.27,61.04 62.43,61.04 61.39,59.99 v60.05,59.99 | 51.21,49.96 49.15,47.9 49.15,43.28 47.47,41.6 47.47,39.65 45.77,37.95 v45.77,35.38 | 51.21,49.96 53.16,51.92 57.99,51.92 61.34,55.27 v62.05,55.27 | v50.52,50.77 51.21,50.09 51.21,49.96
RED  (via drill 0.6)
  Top 0.254: v32.87,30.2 33.1,30.2 33.47,30.57 | v31.37,25.25 31.37,28.19 31.39,28.22
  Top 0.406: RELAY.P$8 25.65,21.21
  Top 2.54: 25.65,21.21 26.09,20.78 v29.77,20.78 30.28,20.78 31.39,21.89 31.39,28.22 31.39,28.5 33.47,30.57 34.04,31.14 34.04,34.98
  Bottom 2.54: 25.65,21.23 26.11,20.78 v29.77,20.78 30.28,20.78 31.39,21.89 31.39,28.5 34.02,31.13 PELTIER.1
RESET  (via drill 0.6)
  Top 0.406: RESET.1 61.54,11.73 64.21,9.07 70.59,9.07 RST.4 | ESP1.1 69.9,62.18 64.97,57.25 v64.64,57.25 | RST.1 71.16,12.5 69.22,12.5 68.34,13.37 ESP3.P$15 67.48,18.71 ESP2.P$15 67.48,24.09 66.19,25.38 61.82,25.38 60.43,26.77 60.43,32.89 59.36,33.96 v59.36,34.87 | R1.2 49.66,60.68 v50.24,60.68
  Bottom 0.406: v59.36,34.87 59.08,35.15 57.53,35.15 55.65,37.03 55.65,38.58 53.11,41.12 53.11,45.36 55.7,47.95 64.75,47.95 65.08,48.28 65.08,56.82 v64.64,57.25 61.32,57.25 57.3,53.24 52.48,53.24 51.61,52.38 48.56,52.38 48.06,52.88 48.06,58.5 v50.24,60.68
  Bottom 1.626: RST.1 RST.4
RXD  (via drill 0.6)
  Top 0.406: ESP3.P$11 60.26,19.91 61.04,19.91 61.48,20.35 ESP2.P$11 61.48,23.13 61.21,23.39 60.66,23.39 58.45,25.6 58.45,30.2 v58.12,30.53 | ESP1.21 67.9,51.15 65.18,53.87 v64.01,53.87
  Bottom 0.406: SERIAL6.3 46.3,15.21 47.6,16.51 56.85,16.51 ESP3.P$11 58.18,21.75 56.44,23.5 53.09,23.5 52.65,23.06 SERIAL4.2 | v64.01,53.87 63.65,53.87 62.08,52.3 62.08,50.24 61.77,49.94 54.56,49.94 51.13,46.51 51.13,40.03 52.98,38.18 52.98,36.52 57.61,31.9 57.61,31.04 v58.12,30.53
SCLK  (via drill 0.6)
  Top 0.406: IC2.P$13 36.13,49.67 37.49,48.31 37.49,46.35 39.8,44.04 46.02,44.04 47.07,43 47.07,38.91 47.52,38.46 50.52,38.46 v50.8,38.73 | ESP3.P$3 68.98,41.33 ESP2.P$3 68.98,37.43 68.02,36.47 52.53,36.47 v51.99,35.94 | ESP1.5 61.9,62.64 61.62,62.36 61.06,62.36 v60.81,62.1
  Bottom 0.406: ESP3.P$3 70.88,44 68.38,46.51 68.38,59.77 66.98,61.16 65.2,61.16 64.01,62.36 61.06,62.36 v60.81,62.1 | v51.99,35.94 51.99,37.54 v50.8,38.73
SDIO  (via drill 0.6)
  Top 0.406: ESP2.P$7 62.98,40.99 ESP3.P$7 59.9,44.06 ESP1.17 59.9,52.01 v59.82,52.09 | v33.07,52.5 33.3,52.5 34.75,51.05 35.55,51.05 IC2.P$14 36.08,50.94 38.15,48.87 38.15,46.66 40.11,44.7 46.43,44.7 47.73,43.41 47.73,40.18 v48.51,39.4 | R3.2 49.23,66.4 v50.37,66.4
  Bottom 0.406: v59.82,52.09 58.98,51.26 53.54,51.26 49.81,47.52 49.81,42.88 48.13,41.2 48.13,39.78 v48.51,39.4 | v33.07,52.5 33.07,56.69 34.82,58.45 40.21,58.45 48.16,66.4 v50.37,66.4
TOUT  (via drill 0.6)
  Top 0.406: ESP1.2 67.9,61.27 64.8,58.17 v62.51,58.17 | ESP3.P$16 68.98,19.75 ESP2.P$16 68.98,23.66 66.6,26.04 62.31,26.04 61.09,27.25 61.09,33.93 60.63,34.39 v60.58,34.39 | R9.1 R10.1 48.82,57.2 49.86,56.16 v50.29,56.16
  Bottom 0.406: v60.58,34.39 60.58,35.43 59.87,36.14 57.63,36.14 56.31,37.47 56.31,38.94 53.77,41.48 53.77,44.98 56.08,47.3 65.05,47.3 65.73,47.98 65.73,57.84 65.41,58.17 v62.51,58.17 61.21,58.17 56.95,53.9 52.17,53.9 51.31,53.03 49.17,53.03 48.72,53.49 48.72,54.59 v50.29,56.16
TXD  (via drill 0.6)
  Top 0.406: ESP3.P$12 62.98,20.09 ESP2.P$12 62.98,23.41 62.33,24.05 61.06,24.05 59.11,26.01 59.11,31.45 v58.7,31.85 | ESP1.22 69.9,50.27 65.28,54.89 63.35,54.89 62.87,54.41 62.87,52.96 63.42,52.4 v63.96,52.4
  Bottom 0.406: SERIAL6.2 48.84,15.21 49.48,15.85 58.73,15.85 ESP3.P$12 60.72,20.28 56.84,24.16 50.72,24.16 50.11,23.55 SERIAL4.3 | v63.96,52.4 63.42,52.4 62.81,51.79 62.81,49.68 62.41,49.28 54.91,49.28 51.79,46.15 51.79,40.41 53.65,38.56 53.65,36.93 58.7,31.88 v58.7,31.85
WELL_TEMP  (via drill 0.6)
  Top 0.406: RL2.2 34.04,64.01 RH.2 32.21,65.84 v30.5,65.84 | v33.07,49.02 32.03,49.02 31.77,49.28 31.77,50.65 31.62,50.8 30.61,50.8 IC2.P$3
  Bottom 0.406: v30.5,65.84 24.61,65.84 24.08,65.3 24.08,49.89 28.6,45.36 30.76,45.36 31.04,45.64 31.04,46.69 32.03,47.68 32.03,48.31 32.74,49.02 v33.07,49.02 33.43,49.02 34.11,48.34 34.11,46.58 34.52,46.18 36.07,46.18 36.32,46.43 36.32,52.48 38.2,54.36 38.79,54.36 39.37,54.94 WELL_TEMP.1

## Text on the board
tPlace: HPWR(WHITE) | HTEMP(PINK) | NinjaPCB ver2.2 | R2 | RT* | WELL / TEMP | R3 | CP1 | R19* | R17* | RH | R20 | R4 | FAN | RL2 | R1 | Q3 | R18 | R22* | RL1 | ^R9 | ^R21 | Q2 | R10 | RD2 | C5 | R15 | R8 | ESP1 / ESP-12 | RD1 | Q1 | R16 | C2 | R5 | R13* | R6 | IC2 | R7 | ^R14 | IC1 | Q6 | C1 | C4 | CP2 | R11 | Q4 | D1 | RED / PELT / BLACK | REG | ESP2 / ESP-WROOM-02 | + | RELAY | DIN4 | C3 | JACK | R12 | D2 | Q5
bPlace: NinjaPCB | SERIAL4 | SERIAL6 | IO0 | M | R | ATX | MODE | RST
tDocu: pipe | lid | well | center | 79 x 73 mm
